FUNCTION "AUTOMATICO" : VOID
TITLE =AUTOMATICO
VERSION : 0.1

BEGIN
NETWORK
TITLE =CONSENSO AL CICLO AUTOMATICO
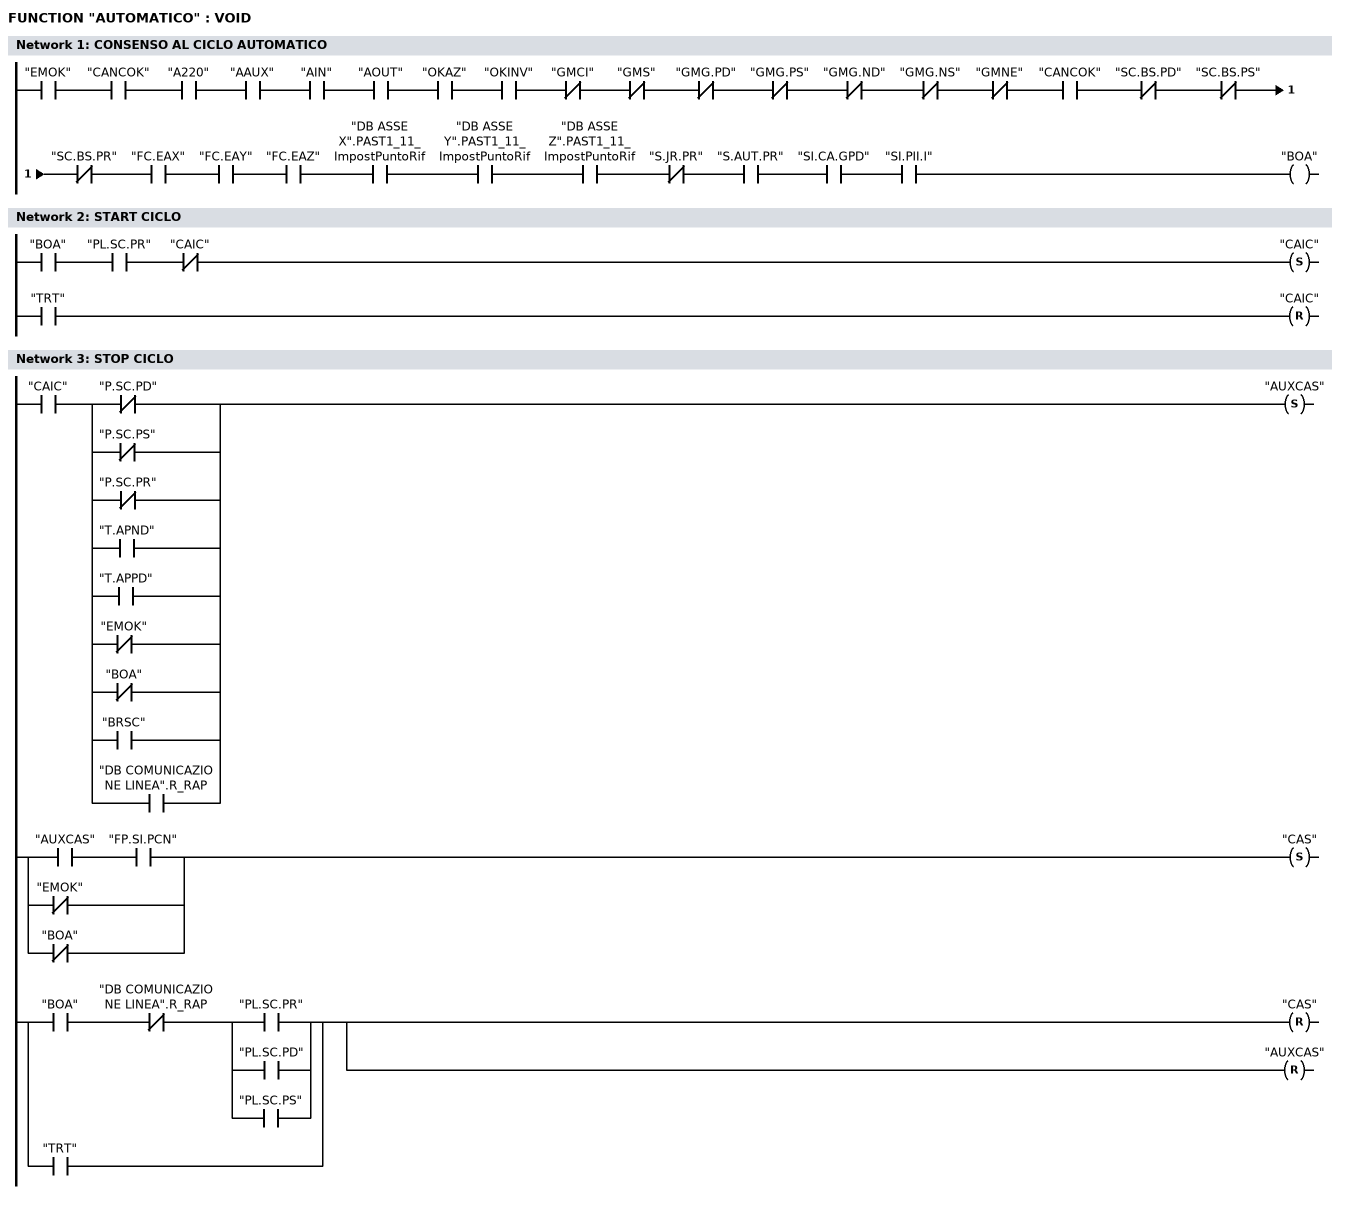
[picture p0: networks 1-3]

      U     "EMOK";
      U     "CANCOK";
      U     "A220";
      U     "AAUX";
      U     "AIN";
      U     "AOUT";
      U     "OKAZ";
      U     "OKINV";
      UN    "GMCI";
//      U     "GMPV"
      UN    "GMS";
      UN    "GMG.PD";
      UN    "GMG.PS";
      UN    "GMG.ND";
      UN    "GMG.NS";
      UN    "GMNE";
      U     "CANCOK";
//      UN(
//      U     "S.IR.PT"
//      U     "IT.A"
//      )
      UN    "SC.BS.PD";
      UN    "SC.BS.PS";
      UN    "SC.BS.PR";
      U     "FC.EAX";
      U     "FC.EAY";
      U     "FC.EAZ";
      U     "DB ASSE X".PAST1_11_ImpostPuntoRif;
      U     "DB ASSE Y".PAST1_11_ImpostPuntoRif;
      U     "DB ASSE Z".PAST1_11_ImpostPuntoRif;
      UN    "S.JR.PR";
      U     "S.AUT.PR";
      U     "SI.CA.GPD";
      U     "SI.PII.I";
      =     "BOA";
NETWORK
TITLE =START CICLO

      U     "BOA";
      U(    ;
      O     "PL.SC.PR";
//      O     "PL.SC.PD"
//      O     "PL.SC.PS"
      )     ;
      UN    "CAIC";
      S     "CAIC";
//===========================
      U     "TRT";
      R     "CAIC";

NETWORK
TITLE =STOP CICLO

      U     "CAIC";
      U(    ;
      ON    "P.SC.PD";
      ON    "P.SC.PS";
      ON    "P.SC.PR";
      O     "T.APND";
      O     "T.APPD";
      ON    "EMOK";
      ON    "BOA";
      O     "BRSC";
      O     "DB COMUNICAZIONE LINEA".R_RAP;
      )     ;
      S     "AUXCAS";
//--------------------------
      U     "AUXCAS";
      U     "FP.SI.PCN";
      ON    "EMOK";
      ON    "BOA";
      S     "CAS";
//=======================================
      U     "BOA";
      UN    "DB COMUNICAZIONE LINEA".R_RAP;
      U(    ;
      O     "PL.SC.PR";
      O     "PL.SC.PD";
      O     "PL.SC.PS";
      )     ;
      O     ;
      U     "TRT";
      R     "CAS";
      R     "AUXCAS";

END_FUNCTION

